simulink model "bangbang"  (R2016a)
settings: Solver=ode4  StartTime=0.0  StopTime=260.0  FixedStep=0.001  RelTol=1e-3
undefined symbols (not defined in the file): gain, initialv, initialy, meansurgeerror, reactiontime, surgethreshold, target

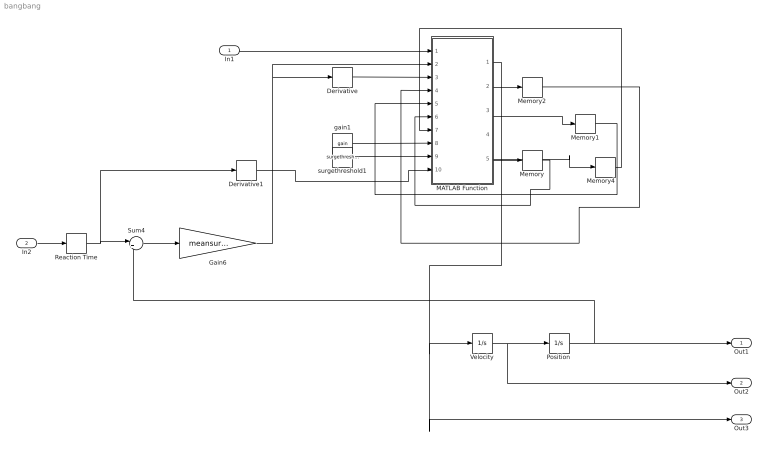
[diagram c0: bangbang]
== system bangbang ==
  In1 : Inport
  In2 : Inport  Port=2
  Derivative : Derivative
  Derivative1 : Derivative
  Gain6 : Gain  Gain=meansurgeerror
  MATLAB Function : MATLAB Function  TreatAsAtomicUnit=on
  Memory{,1..2,4} (4 alike) : Memory
  Position : Integrator  InitialCondition=initialy
  Reaction Time : TransportDelay  DelayTime=reactiontime  InitialOutput=target(1)
  Sum4 : Sum  Inputs=|+-
  Velocity : Integrator  InitialCondition=initialv
  gain1 : Constant  Value=gain
  surgethreshold1 : Constant  Value=surgethreshold
  Out1 : Outport
  Out2 : Outport  Port=2
  Out3 : Outport  Port=3
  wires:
  In1/1 -> MATLAB Function/1(time)
  MATLAB Function/4(newtswitch) -> Memory/1
  Memory/1 -> MATLAB Function/6(tswitch)
  MATLAB Function/3(newt0) -> Memory1/1
  Memory1/1 -> MATLAB Function/5(t0)
  MATLAB Function/2(newlocked) -> Memory2/1
  gain1/1 -> MATLAB Function/8(a_max)
  surgethreshold1/1 -> MATLAB Function/9(surgethreshold)
  Velocity/1 -> Out2/1, Position/1
  MATLAB Function/1(aout) -> Out3/1, Velocity/1
  Gain6/1 -> MATLAB Function/2(e), Derivative/1
  Derivative/1 -> MATLAB Function/3(edot)
  In2/1 -> Reaction Time/1
  MATLAB Function/5(newtstop) -> Memory4/1
  Memory4/1 -> MATLAB Function/7(tstop)
  Memory2/1 -> MATLAB Function/4(locked)
  Derivative1/1 -> MATLAB Function/10(tdot)
  Position/1 -> Out1/1, Sum4/2
  Sum4/1 -> Gain6/1
  Reaction Time/1 -> Derivative1/1, Sum4/1

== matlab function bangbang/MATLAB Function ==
function [aout,newlocked, newt0, newtswitch, newtstop]  = fcn(time,e, edot, locked,t0,tswitch, tstop, a_max, surgethreshold,tdot)
newt0 = t0;
newtswitch = tswitch;
newtstop = tstop;
newlocked = locked;
aout=0;%k1*e; % activate local control law if no other conditions met

a_1 = 1.0;      % constant for abs error weight
a_2 = 0.01;     % constant for abs error derivative weight

if locked ~= 0 
    if time-t0 < tswitch 
       aout = locked*a_max; % first bang
    elseif time-t0 < tstop
       aout = -locked*a_max; % second bang
    else
       newlocked = 0;       % end of bang-bang. Unlock
    end
elseif (a_1*abs(e)+a_2*abs(edot) > surgethreshold && abs(tdot)<1)          % threshold below which surge model is used
    if e == -edot*abs(edot)/(2*a_max)
        f0 = sign(edot);                            % eqn (11)
    else
        f0 = sign(edot*abs(edot)/(2*a_max) + e);    % eqn (9) & (10) of Costello
    end
  %  if f0 == sign(edot) % eqn (13) in Costello doesn't really make sense -
                         %  would need to set a flag that e == -edot*abs(edot)/(2*a_max)
   %     newtswitch = 0;
  % else
        
        newtswitch = (sqrt(0.5*(edot/(a_max*f0)).^2+ e/(a_max*f0)) ...
                     + edot/(a_max*f0)); % eqn (12) from Costello
   % end
        
    newlocked = f0;    % lock, and give information about direction of error which is fed back
    
    newt0=time;             % remember start of bang-bang 
    newtstop = newtswitch + (sqrt(0.5*(edot/(a_max*f0)).^2 + e/(a_max*f0))); %
    aout = newlocked*a_max;
end
